| IBIS file stm32u3b5_3c5_lqfp144.ibs
[IBIS ver] 4.2
[File name] stm32u3b5_3c5_lqfp144.ibs
[File Rev] 0.1
[Date] 09-03-2026
[Source] Data Created at STMicroelectronics
[Notes]  File originated from ELDO simulations.
[Disclaimer]  This information is for modeling purpose only and is
   not guaranted. The information is subject to change without
   notice.
[Copyright] Copyright 2026 STMicroelectronics Inc.
|   Component stm32u3b5_3c5_lqfp144
[Component] stm32u3b5_3c5_lqfp144
[Manufacturer] STMicroelectronics
[Package]
| variable   typ   min   max
R_pkg  0  NA  NA
L_pkg  0  NA  NA
C_pkg  0  NA  NA
[Pin]   signal_name   model_name
1  PE2  io8_ft_100m
2  PE3  io8_ft_100m_hslv
3  PE4  io8_ft_100m
4  PE5  io8_ft_100m
5  PE6  io8_ft_100m
6  VBAT  power
7  PC13  io8_ft_100m_v33
8  PC14-OSC32_IN  io_ft_tamp
9  PC15-OSC32_OUT  io_ft_tamp
10  PF0  io8_ft_100m_hslv
11  PF1  io8_ft_100m_hslv
12  PF2  io8_ft_100m
13  PF3  io8_ft_100m
14  PF4  io8_ft_100m
15  PF5  io8_ft_100m
16  VSS  gnd
17  VDD  power
18  PF6  io8_ft_100m_hslv
19  PF7  io8_ft_100m_hslv
20  PF8  io8_ft_100m_hslv
21  PF9  io8_ft_100m_hslv
22  PF10  io8_ft_100m_hslv
23  PH0-OSC_IN  io8_ft_100m
24  PH1-OSC_OUT  io8_ft_100m
25  NRST  ioreset_v33
26  PC0  io8_ft_100m_hslv
27  PC1  io8_ft_100m_hslv
28  PC2  io8_ft_100m_hslv
29  PC3  io8_ft_100m_hslv
30  VSSA  nc
31  VREFM  nc
32  VREFP  nc
33  VDDA  nc
34  PA0  io8_ft_100m
35  PA1  io8_ft_100m_hslv
36  PA2  io8_ft_100m_hslv
37  PA3  io8_ft_100m_hslv
38  VSS  gnd
39  VDD  power
40  PA4  io8_ft_100m_hslv
41  PA5  io8_ft_100m
42  PA6  io8_ft_100m_hslv
43  PA7  io8_ft_100m_hslv
44  PC4  io8_ft_100m_hslv
45  PC5  io8_ft_100m
46  PB0  io8_ft_100m_hslv
47  PB1  io8_ft_100m_hslv
48  PB2  io8_ft_100m_hslv
49  PF11  io8_ft_100m_hslv
50  PF12  io8_ft_100m
51  VSS  gnd
52  VDD  power
53  PF13  io8_ft_100m
54  PF14  io8_ft_100m_hslv
55  PF15  io8_ft_100m_hslv
56  PG0  io8_ft_100m
57  PG1  io8_ft_100m
58  PE7  io8_ft_100m
59  PE8  io8_ft_100m
60  PE9  io8_ft_100m_hslv
61  VSS  gnd
62  VDD  power
63  PE10  io8_ft_100m_hslv
64  PE11  io8_ft_100m_hslv
65  PE12  io8_ft_100m_hslv
66  PE13  io8_ft_100m_hslv
67  PE14  io8_ft_100m_hslv
68  PE15  io8_ft_100m_hslv
69  PB10  io8_ft_100m_hslv
70  VCAP  nc
71  VSS  gnd
72  VDD  power
73  PB12  io8_ft_100m_hslv
74  PB13  io8_ft_100m_hslv
75  PB14  io8_ft_100m_hslv
76  PB15  io8_ft_100m
77  PD8  io8_ft_100m
78  PD9  io8_ft_100m
79  PD10  io8_ft_100m
80  PD11  io8_ft_100m_hslv
81  PD12  io8_ft_100m_hslv
82  PD13  io8_ft_100m_hslv
83  VSS  gnd
84  VDD  power
85  PD14  io8_ft_100m
86  PD15  io8_ft_100m
87  PG2  io8_ft_100m_hslv
88  PG3  io8_ft_100m_hslv
89  PG4  io8_ft_100m_hslv
90  PG5  io8_ft_100m_hslv
91  PG6  io8_ft_100m_hslv
92  PG7  io8_ft_100m_hslv
93  PG8  io8_ft_100m_hslv
94  VSS  gnd
95  VDDIO2  power
96  PC6  io8_ft_100m_hslv
97  PC7  io8_ft_100m_hslv
98  PC8  io8_ft_100m_hslv
99  PC9  io8_ft_100m_hslv
100  PA8  io8_ft_100m_hslv
101  PA9  io8_ft_100m
102  PA10  io8_ft_100m
103  PA11  io8usb_ft_phy
104  PA12  io8usb_ft_phy
105  PA13  io8_ft_100m
106  VDDUSB  power
107  VSS  gnd
108  VDD  power
109  PA14  io8_ft_100m
110  PA15  io8_ft_100m
111  PC10  io8_ft_100m_hslv
112  PC11  io8_ft_100m_hslv
113  PC12  io8_ft_100m_hslv
114  PD0  io8_ft_100m
115  PD1  io8_ft_100m
116  PD2  io8_ft_100m_hslv
117  PD3  io8_ft_100m_hslv
118  PD4  io8_ft_100m_hslv
119  PD5  io8_ft_100m_hslv
120  VSS  gnd
121  VDD  power
122  PD6  io8_ft_100m_hslv
123  PD7  io8_ft_100m_hslv
124  PG9  io8_ft_100m_hslv
125  PG10  io8_ft_100m_hslv
126  PG11  io8_ft_100m_hslv
127  PG12  io8_ft_100m_hslv
128  PG13  io8_ft_100m_hslv
129  PG14  io8_ft_100m_hslv
130  VSS  gnd
131  VDDIO2  power
132  PG15  io8_ft_100m_hslv
133  PB3  io8_ft_100m_hslv
134  PB4  io8_ft_100m_hslv
135  PB5  io8_ft_100m_hslv
136  PB6  io8_ft_100m_hslv
137  PB7  io8_ft_100m_hslv
138  PH3-BOOT0  io8_ft_100m_hslv
139  PB8  io8_ft_100m_hslv
140  PB9  io8_ft_100m_hslv
141  PE0  io8_ft_100m
142  PE1  io8_ft_100m
143  VSS  gnd
144  VDD  power
[Package Model]   42a-lqfp-20x20-144-251212
[Pin Mapping]   pulldown_ref   pullup_ref   | Comment
1  gndio  vddio
2  gndio  vddio
3  gndio  vddio
4  gndio  vddio
5  gndio  vddio
6  nc  vsw
7  gndio  vsw
8  gndio  vsw
9  gndio  vsw
10  gndio  vddio
11  gndio  vddio
12  gndio  vddio
13  gndio  vddio
14  gndio  vddio
15  gndio  vddio
16  gndio  nc
17  nc  vddio
18  gndio  vddio
19  gndio  vddio
20  gndio  vddio
21  gndio  vddio
22  gndio  vddio
23  gndio  vddio
24  gndio  vddio
25  gndio  vddio
26  gndio  vddio
27  gndio  vddio
28  gndio  vddio
29  gndio  vddio
30  nc  nc
31  nc  nc
32  nc  nc
33  nc  nc
34  gndio  vddio
35  gndio  vddio
36  gndio  vddio
37  gndio  vddio
38  gndio  nc
39  nc  vddio
40  gndio  vddio
41  gndio  vddio
42  gndio  vddio
43  gndio  vddio
44  gndio  vddio
45  gndio  vddio
46  gndio  vddio
47  gndio  vddio
48  gndio  vddio
49  gndio  vddio
50  gndio  vddio
51  gndio  nc
52  nc  vddio
53  gndio  vddio
54  gndio  vddio
55  gndio  vddio
56  gndio  vddio
57  gndio  vddio
58  gndio  vddio
59  gndio  vddio
60  gndio  vddio
61  gndio  nc
62  nc  vddio
63  gndio  vddio
64  gndio  vddio
65  gndio  vddio
66  gndio  vddio
67  gndio  vddio
68  gndio  vddio
69  gndio  vddio
70  nc  nc
71  gndio  nc
72  nc  vddio
73  gndio  vddio
74  gndio  vddio
75  gndio  vddio
76  gndio  vddio
77  gndio  vddio
78  gndio  vddio
79  gndio  vddio
80  gndio  vddio
81  gndio  vddio
82  gndio  vddio
83  gndio  nc
84  nc  vddio
85  gndio  vddio
86  gndio  vddio
87  gndio  vddio2
88  gndio  vddio2
89  gndio  vddio2
90  gndio  vddio2
91  gndio  vddio2
92  gndio  vddio2
93  gndio  vddio2
94  gndio  nc
95  nc  vddio2
96  gndio  vddio
97  gndio  vddio
98  gndio  vddio
99  gndio  vddio
100  gndio  vddio
101  gndio  vddio
102  gndio  vddio
103  gndio  vddusb  | Depending on IO usage
| 103  gndio  vddio  | Depending on IO usage
104  gndio  vddusb  | Depending on IO usage
| 104  gndio  vddio  | Depending on IO usage
105  gndio  vddio
106  nc  vddusb
107  gndio  nc
108  nc  vddio
109  gndio  vddio
110  gndio  vddio
111  gndio  vddio
112  gndio  vddio
113  gndio  vddio
114  gndio  vddio
115  gndio  vddio
116  gndio  vddio
117  gndio  vddio
118  gndio  vddio
119  gndio  vddio
120  gndio  nc
121  nc  vddio
122  gndio  vddio
123  gndio  vddio
124  gndio  vddio2
125  gndio  vddio2
126  gndio  vddio2
127  gndio  vddio2
128  gndio  vddio2
129  gndio  vddio2
130  gndio  nc
131  nc  vddio2
132  gndio  vddio2
133  gndio  vddio
134  gndio  vddio
135  gndio  vddio
136  gndio  vddio
137  gndio  vddio
138  gndio  vddio
139  gndio  vddio
140  gndio  vddio
141  gndio  vddio
142  gndio  vddio
143  gndio  nc
144  nc  vddio
|[Diff Pin]  inv_pin  vdiff  tdelay_typ  tdelay_min  tdelay_max
|104  103  NA  NA  NA  NA
[Model Selector] io8_ft_100m
io8_ft_100m_ls_1v2  "GPIO 100MHz - 5V tolerant - low speed - 1.2V range"
io8_ft_100m_ls_1v8  "GPIO 100MHz - 5V tolerant - low speed - 1.8V range"
io8_ft_100m_ls_3v3  "GPIO 100MHz - 5V tolerant - low speed - 3.3V range"
io8_ft_100m_ms_1v2  "GPIO 100MHz - 5V tolerant - med speed - 1.2V range"
io8_ft_100m_ms_1v8  "GPIO 100MHz - 5V tolerant - med speed - 1.8V range"
io8_ft_100m_ms_3v3  "GPIO 100MHz - 5V tolerant - med speed - 3.3V range"
io8_ft_100m_fs_1v2  "GPIO 100MHz - 5V tolerant - fast speed - 1.2V range"
io8_ft_100m_fs_1v8  "GPIO 100MHz - 5V tolerant - fast speed - 1.8V range"
io8_ft_100m_fs_3v3  "GPIO 100MHz - 5V tolerant - fast speed - 3.3V range"
io8_ft_100m_hs_1v2  "GPIO 100MHz - 5V tolerant - high speed - 1.2V range"
io8_ft_100m_hs_1v8  "GPIO 100MHz - 5V tolerant - high speed - 1.8V range"
io8_ft_100m_hs_3v3  "GPIO 100MHz - 5V tolerant - high speed - 3.3V range"
[Model Selector] io8_ft_100m_hslv
io8_ft_100m_ls_1v2  "GPIO 100MHz - 5V tolerant - low speed - 1.2V range"
io8_ft_100m_ls_1v8  "GPIO 100MHz - 5V tolerant - low speed - 1.8V range"
io8_ft_100m_ls_3v3  "GPIO 100MHz - 5V tolerant - low speed - 3.3V range"
io8_ft_100m_ms_1v2  "GPIO 100MHz - 5V tolerant - med speed - 1.2V range"
io8_ft_100m_ms_1v8  "GPIO 100MHz - 5V tolerant - med speed - 1.8V range"
io8_ft_100m_ms_3v3  "GPIO 100MHz - 5V tolerant - med speed - 3.3V range"
io8_ft_100m_fs_1v2  "GPIO 100MHz - 5V tolerant - fast speed - 1.2V range"
io8_ft_100m_fs_1v8  "GPIO 100MHz - 5V tolerant - fast speed - 1.8V range"
io8_ft_100m_fs_3v3  "GPIO 100MHz - 5V tolerant - fast speed - 3.3V range"
io8_ft_100m_hs_1v2  "GPIO 100MHz - 5V tolerant - high speed - 1.2V range"
io8_ft_100m_hs_1v8  "GPIO 100MHz - 5V tolerant - high speed - 1.8V range"
io8_ft_100m_hs_3v3  "GPIO 100MHz - 5V tolerant - high speed - 3.3V range"
io8_ft_100m_hslv_ls_1v2  "GPIO 100MHz low voltage optimization - 5V tolerant - low speed - 1.2V range"
io8_ft_100m_hslv_ls_1v8  "GPIO 100MHz low voltage optimization - 5V tolerant - low speed - 1.8V range"
io8_ft_100m_hslv_ls_2v5  "GPIO 100MHz low voltage optimization - 5V tolerant - low speed - 3.3V range"
io8_ft_100m_hslv_ms_1v2  "GPIO 100MHz low voltage optimization - 5V tolerant - med speed - 1.2V range"
io8_ft_100m_hslv_ms_1v8  "GPIO 100MHz low voltage optimization - 5V tolerant - med speed - 1.8V range"
io8_ft_100m_hslv_ms_2v5  "GPIO 100MHz low voltage optimization - 5V tolerant - med speed - 3.3V range"
io8_ft_100m_hslv_fs_1v2  "GPIO 100MHz low voltage optimization - 5V tolerant - fast speed - 1.2V range"
io8_ft_100m_hslv_fs_1v8  "GPIO 100MHz low voltage optimization - 5V tolerant - fast speed - 1.8V range"
io8_ft_100m_hslv_fs_2v5  "GPIO 100MHz low voltage optimization - 5V tolerant - fast speed - 3.3V range"
io8_ft_100m_hslv_hs_1v2  "GPIO 100MHz low voltage optimization - 5V tolerant - high speed - 1.2V range"
io8_ft_100m_hslv_hs_1v8  "GPIO 100MHz low voltage optimization - 5V tolerant - high speed - 1.8V range"
io8_ft_100m_hslv_hs_2v5  "GPIO 100MHz low voltage optimization - 5V tolerant - high speed - 3.3V range"
[Model Selector] io8_ft_100m_v33
io8_ft_100m_v33_ls_1v2  "GPIO_V33 100MHz - 5V tolerant - low speed - 1.2V range"
io8_ft_100m_v33_ls_1v8  "GPIO_V33 100MHz - 5V tolerant - low speed - 1.8V range"
io8_ft_100m_v33_ls_3v3  "GPIO_V33 100MHz - 5V tolerant - low speed - 3.3V range"
io8_ft_100m_v33_ms_1v2  "GPIO_V33 100MHz - 5V tolerant - med speed - 1.2V range"
io8_ft_100m_v33_ms_1v8  "GPIO_V33 100MHz - 5V tolerant - med speed - 1.8V range"
io8_ft_100m_v33_ms_3v3  "GPIO_V33 100MHz - 5V tolerant - med speed - 3.3V range"
io8_ft_100m_v33_fs_1v2  "GPIO_V33 100MHz - 5V tolerant - fast speed - 1.2V range"
io8_ft_100m_v33_fs_1v8  "GPIO_V33 100MHz - 5V tolerant - fast speed - 1.8V range"
io8_ft_100m_v33_fs_3v3  "GPIO_V33 100MHz - 5V tolerant - fast speed - 3.3V range"
io8_ft_100m_v33_hs_1v2  "GPIO_V33 100MHz - 5V tolerant - high speed - 1.2V range"
io8_ft_100m_v33_hs_1v8  "GPIO_V33 100MHz - 5V tolerant - high speed - 1.8V range"
io8_ft_100m_v33_hs_3v3  "GPIO_V33 100MHz - 5V tolerant - high speed - 3.3V range"
[Model Selector] io8usb_ft_phy
io8_ft_100m_ls_1v2  "GPIO 100MHz - 5V tolerant - low speed - 1.2V range"
io8_ft_100m_ls_1v8  "GPIO 100MHz - 5V tolerant - low speed - 1.8V range"
io8_ft_100m_ls_3v3  "GPIO 100MHz - 5V tolerant - low speed - 3.3V range"
io8_ft_100m_ms_1v2  "GPIO 100MHz - 5V tolerant - med speed - 1.2V range"
io8_ft_100m_ms_1v8  "GPIO 100MHz - 5V tolerant - med speed - 1.8V range"
io8_ft_100m_ms_3v3  "GPIO 100MHz - 5V tolerant - med speed - 3.3V range"
io8_ft_100m_fs_1v2  "GPIO 100MHz - 5V tolerant - fast speed - 1.2V range"
io8_ft_100m_fs_1v8  "GPIO 100MHz - 5V tolerant - fast speed - 1.8V range"
io8_ft_100m_fs_3v3  "GPIO 100MHz - 5V tolerant - fast speed - 3.3V range"
io8_ft_100m_hs_1v2  "GPIO 100MHz - 5V tolerant - high speed - 1.2V range"
io8_ft_100m_hs_1v8  "GPIO 100MHz - 5V tolerant - high speed - 1.8V range"
io8_ft_100m_hs_3v3  "GPIO 100MHz - 5V tolerant - high speed - 3.3V range"
io8usb_ft_phy_hs_3v3   "USB full speed"
io8usb_ft_phy_ls_3v3   "USB low speed"
[Model Selector] io_ft_tamp
io_ft_tamp_ls_1v2 "io8_ft tamp low speed @ 1.2V"
io_ft_tamp_ls_1v8 "io8_ft tamp low speed @ 1.8V"
io_ft_tamp_ls_3v3 "io8_ft tamp low speed @ 3.3V"
io_ft_tamp_ms_1v2 "io8_ft tamp med speed @ 1.2V"
io_ft_tamp_ms_1v8 "io8_ft tamp med speed @ 1.8V"
io_ft_tamp_ms_3v3 "io8_ft tamp med speed @ 3.3V"
io_ft_tamp_fs_1v2 "io8_ft tamp fast speed @ 1.2V"
io_ft_tamp_fs_1v8 "io8_ft tamp fast speed @ 1.8V"
io_ft_tamp_fs_3v3 "io8_ft tamp fast speed @ 3.3V"
io_ft_tamp_hs_1v2 "io8_ft tamp high speed @ 1.2V"
io_ft_tamp_hs_1v8 "io8_ft tamp high speed @ 1.8V"
io_ft_tamp_hs_3v3 "io8_ft tamp high speed @ 3.3V"
[Model Selector] ioreset_v33
ioreset_v33_1v2 "Reset PAD. 5V tolerant. 1.2V range"
ioreset_v33_1v8 "Reset PAD. 5V tolerant. 1.8V range"
ioreset_v33_3v3 "Reset PAD. 5V tolerant. 3.3V range"
[Define Package Model]  42a-lqfp-20x20-144-251212
[Manufacturer]  Unknown
[OEM]  Unknown
[Description]  None
[Number Of Pins]  139
[Pin Numbers]
| Pin Num   Terminal Name
25 | NRST
34 | PA0
35 | PA1
36 | PA2
37 | PA3
40 | PA4
41 | PA5
42 | PA6
43 | PA7
100 | PA8
101 | PA9
102 | PA10
103 | PA11
104 | PA12
105 | PA13
109 | PA14
110 | PA15
46 | PB0
47 | PB1
48 | PB2
133 | PB3
134 | PB4
135 | PB5
136 | PB6
137 | PB7
139 | PB8
140 | PB9
69 | PB10
73 | PB12
74 | PB13
75 | PB14
76 | PB15
26 | PC0
27 | PC1
28 | PC2
29 | PC3
44 | PC4
45 | PC5
96 | PC6
97 | PC7
98 | PC8
99 | PC9
111 | PC10
112 | PC11
113 | PC12
7 | PC13
8 | PC14-OSC32_IN
9 | PC15-OSC32_OUT
114 | PD0
115 | PD1
116 | PD2
117 | PD3
118 | PD4
119 | PD5
122 | PD6
123 | PD7
77 | PD8
78 | PD9
79 | PD10
80 | PD11
81 | PD12
82 | PD13
85 | PD14
86 | PD15
141 | PE0
142 | PE1
1 | PE2
2 | PE3
3 | PE4
4 | PE5
5 | PE6
58 | PE7
59 | PE8
60 | PE9
63 | PE10
64 | PE11
65 | PE12
66 | PE13
67 | PE14
68 | PE15
10 | PF0
11 | PF1
12 | PF2
13 | PF3
14 | PF4
15 | PF5
18 | PF6
19 | PF7
20 | PF8
21 | PF9
22 | PF10
49 | PF11
50 | PF12
53 | PF13
54 | PF14
55 | PF15
56 | PG0
57 | PG1
87 | PG2
88 | PG3
89 | PG4
90 | PG5
91 | PG6
92 | PG7
93 | PG8
124 | PG9
125 | PG10
126 | PG11
127 | PG12
128 | PG13
129 | PG14
132 | PG15
23 | PH0-OSC_IN
24 | PH1-OSC_OUT
138 | PH3-BOOT0
6 | VBAT
70 | VCAP
17 | VDD
39 | VDD
52 | VDD
62 | VDD
72 | VDD
84 | VDD
108 | VDD
121 | VDD
144 | VDD
33 | VDDA
95 | VDDIO2
131 | VDDIO2
106 | VDDUSB
31 | VREFM
32 | VREFP
16 | VSS
51 | VSS
83 | VSS
94 | VSS
120 | VSS
130 | VSS
30 | VSSA
|[Merged Pins]  16
|38  |  VSS
|61  |  VSS
|71  |  VSS
|107  |  VSS
|143  |  VSS
[Model Data]
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[End Model Data]
[End Package Model]
|End [Component]
| Models and submodels in the file (53): io8_ft_100m_fs_1v2 (I/O), io8_ft_100m_fs_1v8 (I/O), io8_ft_100m_fs_3v3 (I/O), io8_ft_100m_hs_1v2 (I/O), io8_ft_100m_hs_1v8 (I/O), io8_ft_100m_hs_3v3 (I/O), io8_ft_100m_hslv_fs_1v2 (I/O), io8_ft_100m_hslv_fs_1v8 (I/O), io8_ft_100m_hslv_fs_2v5 (I/O), io8_ft_100m_hslv_hs_1v2 (I/O), io8_ft_100m_hslv_hs_1v8 (I/O), io8_ft_100m_hslv_hs_2v5 (I/O), io8_ft_100m_hslv_ls_1v2 (I/O), io8_ft_100m_hslv_ls_1v8 (I/O), io8_ft_100m_hslv_ls_2v5 (I/O), io8_ft_100m_hslv_ms_1v2 (I/O), io8_ft_100m_hslv_ms_1v8 (I/O), io8_ft_100m_hslv_ms_2v5 (I/O), io8_ft_100m_ls_1v2 (I/O), io8_ft_100m_ls_1v8 (I/O), io8_ft_100m_ls_3v3 (I/O), io8_ft_100m_ms_1v2 (I/O), io8_ft_100m_ms_1v8 (I/O), io8_ft_100m_ms_3v3 (I/O), io8_ft_100m_v33_fs_1v2 (I/O), io8_ft_100m_v33_fs_1v8 (I/O), io8_ft_100m_v33_fs_3v3 (I/O), io8_ft_100m_v33_hs_1v2 (I/O), io8_ft_100m_v33_hs_1v8 (I/O), io8_ft_100m_v33_hs_3v3 (I/O), io8_ft_100m_v33_ls_1v2 (I/O), io8_ft_100m_v33_ls_1v8 (I/O), io8_ft_100m_v33_ls_3v3 (I/O), io8_ft_100m_v33_ms_1v2 (I/O), io8_ft_100m_v33_ms_1v8 (I/O), io8_ft_100m_v33_ms_3v3 (I/O), io8usb_ft_phy_hs_3v3 (I/O), io8usb_ft_phy_ls_3v3 (I/O), io_ft_tamp_fs_1v2 (I/O), io_ft_tamp_fs_1v8 (I/O), io_ft_tamp_fs_3v3 (I/O), io_ft_tamp_hs_1v2 (I/O), io_ft_tamp_hs_1v8 (I/O), io_ft_tamp_hs_3v3 (I/O), io_ft_tamp_ls_1v2 (I/O), io_ft_tamp_ls_1v8 (I/O), io_ft_tamp_ls_3v3 (I/O), io_ft_tamp_ms_1v2 (I/O), io_ft_tamp_ms_1v8 (I/O), io_ft_tamp_ms_3v3 (I/O), ioreset_v33_1v2 (I/O_open_drain), ioreset_v33_1v8 (I/O_open_drain), ioreset_v33_3v3 (I/O_open_drain)
